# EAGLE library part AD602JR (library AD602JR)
IC OPAMP VGA 35MHZ 16SOIC Source: Datasheet
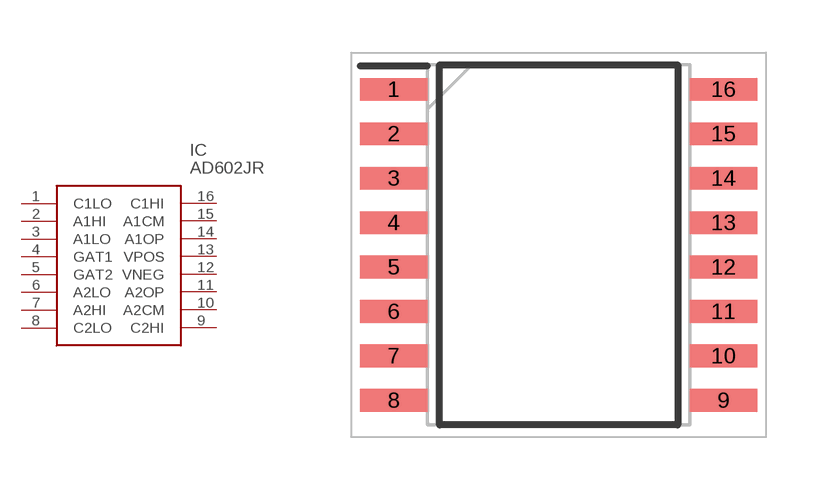
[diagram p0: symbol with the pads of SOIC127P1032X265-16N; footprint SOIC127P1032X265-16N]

Designator prefix IC

## AD602JR (Description: IC OPAMP VGA 35MHZ 16SOIC; Height: 2.65mm; Manufacturer_Name: Analog Devices; Manufacturer_Part_Number: AD602JR)  [SOIC127P1032X265-16N]
1  C1LO
2  A1HI
3  A1LO
4  GAT1
5  GAT2
6  A2LO
7  A2HI
8  C2LO
9  C2HI
10  A2CM
11  A2OP
12  VNEG
13  VPOS
14  A1OP
15  A1CM
16  C1HI

## Footprint SOIC127P1032X265-16N (pad centres in mm)
RW-16 (SOIC)
smd 1.925 x 0.65: 1 -4.712,4.445; 2 -4.712,3.175; 3 -4.712,1.905; 4 -4.712,0.635; 5 -4.712,-0.635; 6 -4.712,-1.905; 7 -4.712,-3.175; 8 -4.712,-4.445; 9 4.712,-4.445; 10 4.712,-3.175; 11 4.712,-1.905; 12 4.712,-0.635; 13 4.712,0.635; 14 4.712,1.905; 15 4.712,3.175; 16 4.712,4.445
